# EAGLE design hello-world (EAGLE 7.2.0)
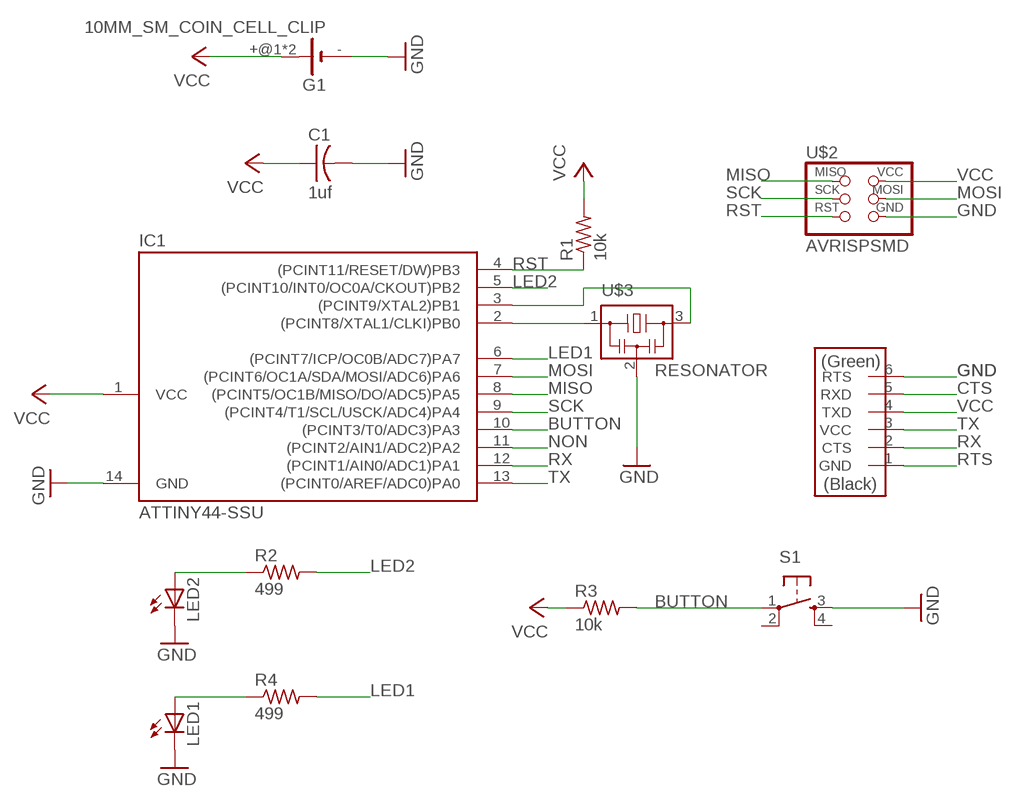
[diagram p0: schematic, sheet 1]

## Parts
C1  1uf  CAP-US1206FAB  [C1206FAB]
G1  10MM_SM_COIN_CELL_CLIP  [10MM_SM_COIN_CELL_CLIP]
IC1  ATTINY44-SSU  [SOIC14]
LED1  LEDSMT1206  [1206]
LED2  LEDSMT1206  [1206]
R1  10k  RES-US1206FAB  [R1206FAB]
R2  499  RES-US1206FAB  [R1206FAB]
R3  10k  RES-US1206FAB  [R1206FAB]
R4  499  RES-US1206FAB  [R1206FAB]
S1  6MM_SWITCH6MM_SWITCH  [6MM_SWITCH]
U$1  FTDI-SMD-HEADER  [1X06SMD]
U$2  AVRISPSMD  [2X03SMD]
U$3  RESONATOR  [EFOBM]

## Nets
BUTTON: IC1.10((PCINT3/T0/ADC3)PA3) R3.2 S1.1(P)
CTS: U$1.5(RXD)
GND: C1.2 G1.- IC1.14(GND) LED1.C LED2.C S1.3(S) U$1.6(RTS) U$2.6(GND) U$3.2
LED1: IC1.6((PCINT7/ICP/OC0B/ADC7)PA7) R4.2
LED2: IC1.5((PCINT10/INT0/OC0A/CKOUT)PB2) R2.2
MISO: IC1.8((PCINT5/OC1B/MISO/DO/ADC5)PA5) U$2.1(MISO)
MOSI: IC1.7((PCINT6/OC1A/SDA/MOSI/ADC6)PA6) U$2.4(MOSI)
N$1: IC1.2((PCINT8/XTAL1/CLKI)PB0) U$3.1
N$12: LED2.A R2.1
N$17: IC1.3((PCINT9/XTAL2)PB1) U$3.3
N$19: LED1.A R4.1
NON: IC1.11((PCINT2/AIN1/ADC2)PA2)
RST: IC1.4((PCINT11/RESET/DW)PB3) R1.1 U$2.5(RST)
RTS: U$1.1(GND)
RX: IC1.12((PCINT1/AIN0/ADC1)PA1) U$1.2(CTS)
SCK: IC1.9((PCINT4/T1/SCL/USCK/ADC4)PA4) U$2.3(SCK)
TX: IC1.13((PCINT0/AREF/ADC0)PA0) U$1.3(VCC)
VCC: C1.1 G1.+@1(+) G1.+@2(+) IC1.1(VCC) R1.2 R3.1 U$1.4(TXD) U$2.2(VCC)
Unconnected: S1.2(P1) S1.4(S1)

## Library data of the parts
C1 = fab:CAP-US
G1 = battery:10MM_SM_COIN_CELL_CLIP: Battery cell clip for CR927
IC1 = fab:ATTINY44
LED1 LED2 = adafruit:LED: LED
R1-R4 = fab:RES-US: Resistor (US Symbol)
S1 = fab:6MM_SWITCH: OMRON SWITCH
U$1 = fab:FTDI-SMD-HEADER
U$2 = fab:AVRISP
U$3 = fab:RESONATOR

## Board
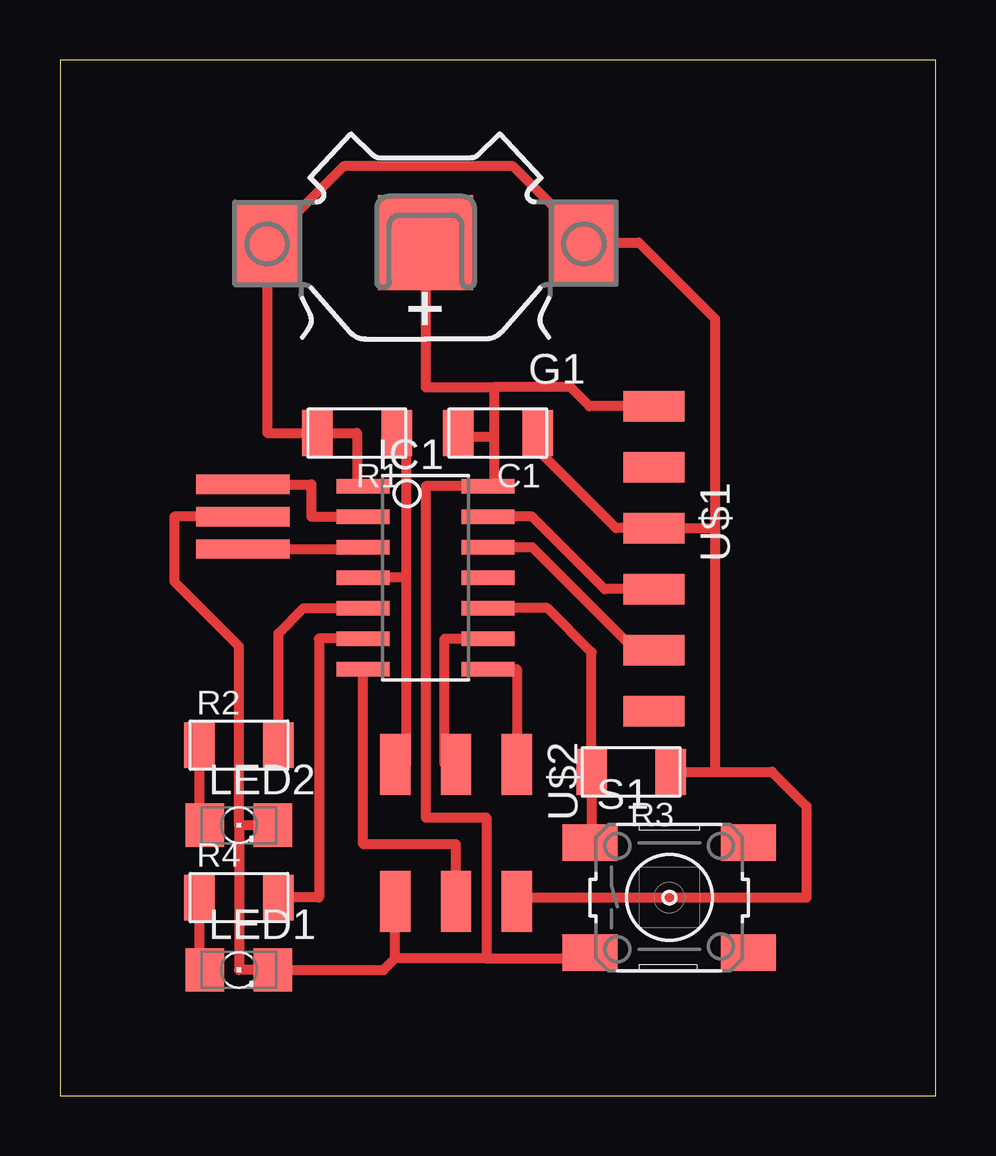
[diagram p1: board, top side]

Size 36.5 x 43.17 mm. Coordinates in mm from the lower left corner, seen from the top.
Outline: 0,0 36.5,0 36.5,43.17 0,43.17 0,0
Copper layers (1*16): Top 0.035mm / dielectric 1.5mm / Bottom 0.035mm
Design rules "default *": minimum track width 10mil, minimum drill 24mil, track to track 16mil, track to pad 16mil, pad to pad 16mil, via to via 16mil, smd to smd 16mil, copper to edge 40mil, drill to drill 8mil, minimum pad ring 10mil, minimum via ring 8mil, stop-mask expansion 4mil, vias tented up to drill 0mil, thermal gap 10mil

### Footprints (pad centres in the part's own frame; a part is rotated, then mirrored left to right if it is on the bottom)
C1206FAB = smd 1.27 x 1.905: 1 -1.651,0; 2 1.651,0
10MM_SM_COIN_CELL_CLIP = smd 2.9 x 3.5: +@1 -6.6,0; +@2 6.6,0 | smd 3.96 x 3.96: - 0,0
SOIC14 = smd 0.61 x 2.21: 1 -3.81,-2.603; 2 -2.54,-2.603; 3 -1.27,-2.603; 4 0,-2.603; 5 1.27,-2.603; 6 2.54,-2.603; 7 3.81,-2.603; 8 3.81,2.603; 9 2.54,2.603; 10 1.27,2.603; 11 0,2.603; 12 -1.27,2.603; 13 -2.54,2.603; 14 -3.81,2.603
1206 = smd 1.6 x 1.803: A -1.422,0; C 1.422,0
R1206FAB = smd 1.27 x 1.905: 1 -1.651,0; 2 1.651,0
6MM_SWITCH = smd 2.286 x 1.524: 1 -3.302,2.286; 2 3.302,2.286; 3 -3.302,-2.286; 4 3.302,-2.286
1X06SMD = smd 2.54 x 1.27: 1 0,6.35; 2 0,3.81; 3 0,1.27; 4 0,-1.27; 5 0,-3.81; 6 0,-6.35
2X03SMD = smd 2.54 x 1.27: 1 -2.857,2.54; 2 2.857,2.54; 3 -2.857,0; 4 2.857,0; 5 -2.857,-2.54; 6 2.857,-2.54
EFOBM = smd 0.8 x 3.9: 1 -1.35,0; 2 0,0; 3 1.35,0

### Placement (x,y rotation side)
C1  18.26,27.62 180 top
G1  15.24,35.56 180 top
IC1  15.24,21.59 270 top
LED1  7.46,5.24 0 top
LED2  7.46,11.27 0 top
R1  12.38,27.62 180 top
R2  7.46,14.61 0 top
R3  23.81,13.49 180 top
R4  7.46,8.26 0 top
S1  25.4,8.26 0 top
U$1  24.77,22.38 180 top
U$2  16.51,10.95 270 top
U$3  7.62,24.13 270 top

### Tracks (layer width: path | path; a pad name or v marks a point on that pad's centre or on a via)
BUTTON
  Top 0.406: IC1.10 20.32,20.32 22.16,18.48 R3.2 22.16,10.6 S1.1
GND
  Top 0.406: U$3.2 4.76,24.13 4.76,21.43 7.46,18.73 7.46,11.27 | 7.46,11.27 7.46,5.24 LED1.C 13.49,5.24 13.97,5.71 | 17.78,5.71 17.78,11.59 15.24,11.59 15.24,25.4 IC1.14 18.1,25.4 18.1,27.46 | 17.78,5.71 13.97,5.71 | 13.97,5.71 U$2.6 | 17.78,5.71 22.23,5.71 22.23,5.97 S1.3 | U$1.6 22.07,28.73 21.27,29.53 18.1,29.53 | 18.1,29.53 18.1,27.46 | LED2.C 7.46,11.27 | C1.2 16.61,27.46 18.1,27.46 | G1.- 15.24,29.53 18.1,29.53
LED1
  Top 0.406: IC1.6 10.79,19.05 10.79,8.26 R4.2
LED2
  Top 0.406: R2.2 9.11,19.27 10.16,20.32 IC1.5
MISO
  Top 0.406: IC1.8 19.05,17.78 U$2.1
MOSI
  Top 0.406: U$2.4 16.51,10.48 12.64,10.48 IC1.7
N$1
  Top 0.406: U$3.1 10.48,25.48 10.48,24.13 IC1.2
N$12
  Top 0.406: R2.1 5.81,11.27 LED2.A
N$17
  Top 0.406: U$3.3 12.64,22.78 IC1.3
N$19
  Top 0.406: R4.1 5.81,4.92 LED1.A
RST
  Top 0.406: 14.45,21.59 IC1.4 | U$2.5 14.45,13.81 14.45,21.59 | 14.45,21.59 14.45,27.62 R1.1
RX
  Top 0.406: IC1.12 19.68,22.86 24.13,18.41 24.61,18.41 U$1.2
SCK
  Top 0.406: U$2.3 16.03,13.81 16.03,19.05 IC1.9
TX
  Top 0.406: U$1.3 22.7,21.11 19.68,24.13 IC1.13
VCC
  Top 0.406: IC1.1 12.38,25.4 12.38,27.62 R1.2 8.64,27.62 G1.+@2 11.81,38.73 18.89,38.73 21.84,35.79 G1.+@1 24.13,35.56 27.3,32.38 27.3,23.65 | R3.1 27.3,13.49 | 27.3,23.65 U$1.4 23.18,23.65 20,26.83 20,27.53 C1.1 | 27.3,23.65 27.3,13.49 | 27.3,13.49 29.69,13.49 31.11,12.06 31.11,8.26 19.05,8.26 U$2.2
